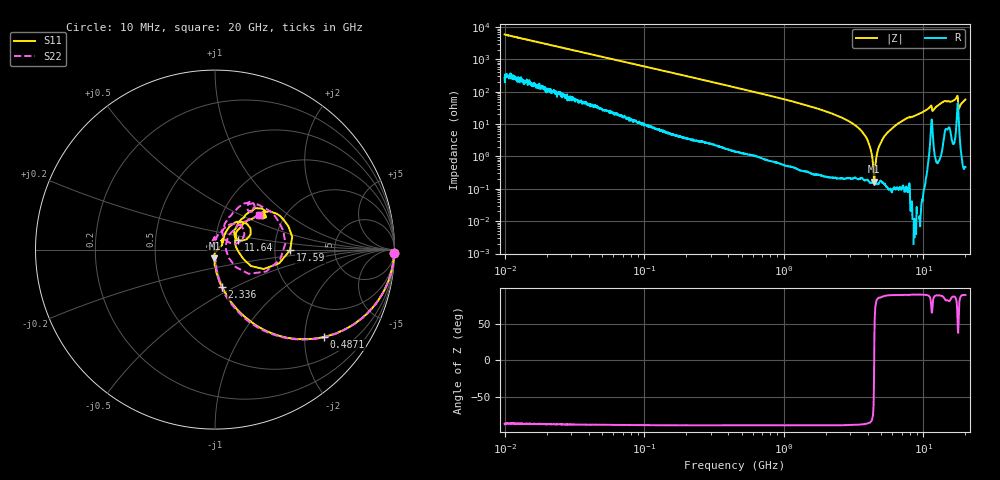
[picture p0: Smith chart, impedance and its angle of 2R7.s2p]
!Keysight Technologies,P5008B,MY61100088,A.16.20.02
!Date: Friday, August 30, 2024 11:18:49
!Correction: S11(C  2-Port  )
!S21(C  2-Port  )
!S12(C  2-Port  )
!S22(C  2-Port  )
!S2P File: Measurements: S11, S21, S12, S22:Log Frequency Sweep
# Hz S  dB  R 50
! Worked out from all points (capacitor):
!   1601 points, 10 MHz to 20 GHz, reference 50 ohm
!   read as one part in series: C = 2.7 pF near 10.39 MHz
!   lowest |Z| = 167 mohm at 4.436 GHz (marker M1)
!   series resonance near 4.443 GHz, so ESL is about 480 pH
!   S11 on the Smith chart (normalised r, x): 10 MHz: open; 487.1 MHz: 1.01, -2.49; 2.336 GHz: 0.99, -0.43; 11.64 GHz: 1.29, +0.14; 17.59 GHz: 2.44, -0.02; 20 GHz: 1.50, +0.64
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1e7  -0.00 -1.0  -35.43 86.3  -35.43 86.4  -0.01 -1.0
3.555162e7  -0.03 -3.4  -24.57 84.9  -24.57 84.9  -0.03 -3.4
1.263918e8  -0.21 -11.8  -13.89 77.4  -13.89 77.4  -0.20 -11.8
4.472136e8  -1.90 -36.3  -4.63 53.0  -4.64 53.0  -1.90 -36.5
4.871375e8  -2.17 -38.7  -4.16 50.6  -4.16 50.6  -2.17 -38.9
1.589917e9  -9.54 -71.2  -0.54 17.9  -0.54 17.9  -9.53 -72.1
2.336087e9  -13.50 -79.4  -0.21 9.6  -0.22 9.6  -13.48 -80.1
3.44879e9  -19.10 -87.6  -0.07 2.1  -0.07 2.1  -18.98 -85.6
4.436224e9  -26.23 -93.8  -0.02 -2.8  -0.02 -2.8  -26.06 -86.5
5.043341e9  -30.17 -98.6  -0.01 -5.3  -0.01 -5.3  -30.18 -82.1
5.652411e9  -36.46 -81.1  0.00 -7.6  0.00 -7.6  -38.44 -95.4
6.012494e9  -38.26 -34.5  0.01 -8.9  0.01 -8.9  -44.35 -164.7
6.643251e9  -30.25 29.1  0.01 -11.1  0.01 -11.1  -31.10 115.3
7.410252e9  -25.03 42.1  0.01 -13.7  0.01 -13.7  -25.52 103.0
8.667956e9  -24.60 55.3  0.02 -17.7  0.01 -17.8  -24.76 83.2
1.099193e10  -15.46 55.5  -0.17 -27.2  -0.17 -27.3  -15.83 59.7
1.163675e10  -17.09 22.4  -0.55 -23.2  -0.55 -23.3  -21.88 42.6
1.393898e10  -9.29 42.0  -0.66 -36.2  -0.66 -36.4  -9.61 53.5
1.7017e10  -8.49 34.1  -0.96 -45.7  -0.97 -45.9  -8.88 39.9
1.75924e10  -7.57 -0.4  -3.53 -41.4  -3.53 -41.6  -8.69 -8.4
1.853616e10  -16.21 39.5  -0.20 -40.2  -0.20 -40.4  -16.79 46.0
2e10  -10.05 37.7  -0.44 -50.9  -0.44 -51.1  -10.11 38.0
